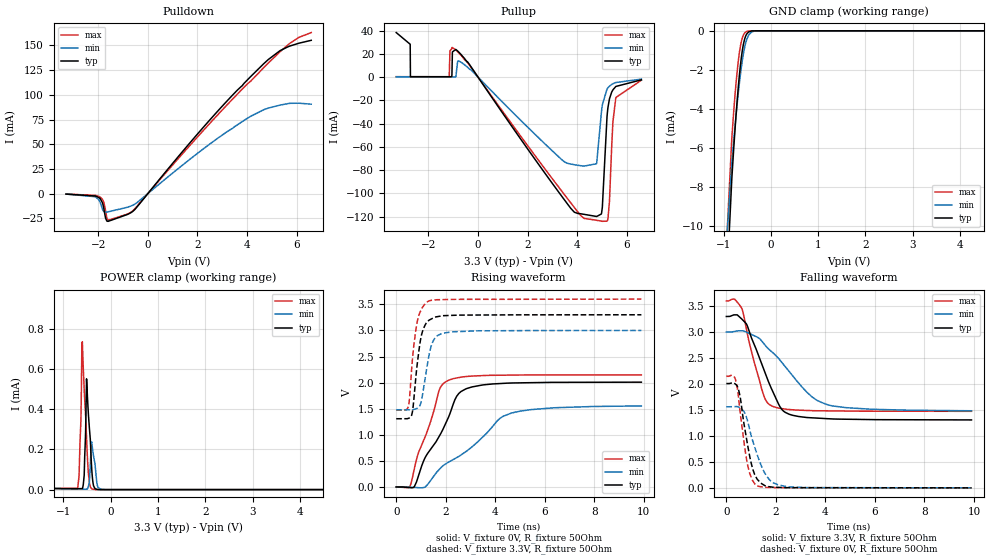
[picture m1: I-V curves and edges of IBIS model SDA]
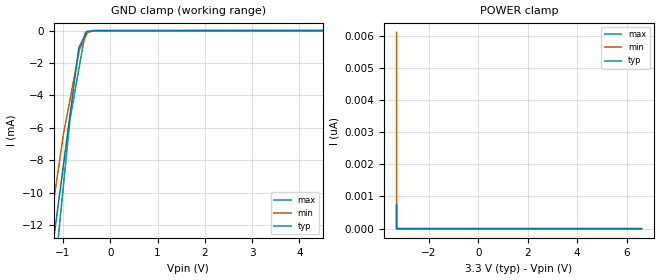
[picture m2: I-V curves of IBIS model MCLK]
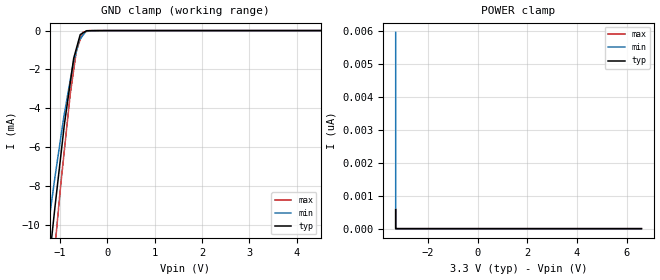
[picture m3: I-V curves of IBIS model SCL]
| Texas Instruments Incorporated
| 25-W STEREO AMPLIFIER WITH EQ, DRC, AND DIRECT-PATH HEADPHONE AMPLIFIER
| Marketing part#   Voltage Range   Package-type   #pins/pkg drawing
| TAS5729MD   3.0V - 3.6V   TQFP   48-pin TQFP
[IBIS Ver]   4.0
[File name]   tas5729md.ibs
[File Rev]   1.0
[Date]   06/06/2012
[Source]   Model built from TISPICED simulations at:
   Texas Instruments Incorporated.
   Analog-eLab, HPA
   12500 TI Blvd
   Dallas, TX -75243
   For Support e-mail: elab_ibis@list.ti.com
[Notes]   Revision History
   Rev 1.0: 06/06/2012
   - ccomp values are based on PVT settings:
   WEAK: Low Voltage, High Temperature, Weak Process
   NOM: Nominal Voltage, Nominal Temperature, Nominal Process
   STRONG: High Voltage, Low Temperature, Fast Process
   - User may change ccomp in the order of number values as
   per end simulator used
   - C_comp although listed in numberical order of value are obtained from varying PVT conditions.
   For PVT conditions for each specific value, refer to the buffer description under repective [Model].
   IBIS model user is responsible for using appropriate C_comp to simulate for Signal Integrity.
   - Non-monotonic behavior in SDA model is a result of simulation.
[Disclaimer] This model is designed as an aid for customers of Texas Instruments.
 TI and its licensors and suppliers make no warranties, either expressed
 or implied, with respect to this  model, including the warranties of
 merchantability or fitness for a particular purpose.
 The model is provided solely on an "as is" basis. The entire risk as to
 its quality and performance is with the customer.
[Copyright] (C)Copyright 2012 Texas Instruments Incorporated.
   All rights reserved.
|   Component TAS5729MD
[Component]   TAS5729MD
[Manufacturer]  Texas Instruments Incorporated
[Package]   |48-pin TQFP PHP package
|   typ   min   max
R_pkg   0.111   0.052   0.195
L_pkg   2.811nH   1.641nH   4.365nH
C_pkg   0.561pF   0.383pF   0.971pF
[Pin] signal_name   model_name   R_pin   L_pin   C_pin
1   GND   GND   0.06305   3.25293nH   0.9711pF
2   OUTA   NC   0.08589   3.49122nH   0.77876pF
3   BSTA   NC   0.16148   3.75361nH   0.72245pF
4   PVDD   POWER   0.06585   2.58699nH   0.74279pF
5   PWM1   NC   0.07479   2.04281nH   0.58008pF
6   PWM2   NC   0.06489   1.79675nH   0.55462pF
7   HPIL   NC   0.06029   1.67272nH   0.54983pF
8   HPOL   NC   0.06108   1.65283nH   0.5297pF
9   HPOR   NC   0.06399   1.64098nH   0.52278pF
10   HPIR   NC   0.06787   1.70652nH   0.54865pF
11   HPVSS   NC   0.07197   1.75312nH   0.54261pF
12   CN   NC   0.14722   2.80415nH   0.40929pF
13   CP   NC   0.16145   3.02753nH   0.43109pF
14   HPVDD   NC   0.17406   3.23001nH   0.45908pF
15   GND   GND   0.06558   2.05127nH   0.44725pF
16   FLTM   NC   0.1246   2.46433nH   0.42269pF
17   FTLP   NC   0.13785   2.72862nH   0.45429pF
18   AVDD_REG1   NC   0.15617   3.04909nH   0.4946pF
19   AVDD   POWER   0.09525   3.06484nH   0.55645pF
20   ADR   SDIN   0.19547   3.8041nH   0.50443pF
21   MCLK   MCLK   0.14557   3.25076nH   0.56537pF
22   ROSC   NC   0.14501   3.50685nH   0.71349pF
23   GND   GND   0.09037   3.53737nH   0.80119pF
24   DVDD_REG   NC   0.10021   4.1032nH   0.7864pF
25   PDN   SDIN   0.15766   4.36474nH   0.75795pF
26   LRCLK   MCLK   0.15465   3.95793nH   0.77612pF
27   SCLK   MCLK   0.1548   3.65915nH   0.72538pF
28   SDIN1   SDIN   0.15922   3.46366nH   0.58952pF
29   SDA   SDA   0.15909   3.2297nH   0.47015pF
30   SCLK   SCL   0.13875   2.82626nH   0.47213pF
31   NC   NC   0.01329   1.07519nH   0.34093pF
32   RESET   NC   0.10958   2.28802nH   0.41439pF
33   TEST   SDIN   0.1143   2.30153nH   0.40259pF
34   DVDD_REG   NC   0.06503   2.0377nH   0.45379pF
35   GND   GND   0.06927   2.14655nH   0.4476pF
36   GND   GND   0.0667   2.76518nH   0.50798pF
37   AVDD_REG2   NC   0.13522   2.61575nH   0.39962pF
38   SSTIMER   NC   0.11443   2.29623nH   0.40178pF
39   HP_SD   SDIN   0.09788   2.05796nH   0.39429pF
40   GVDD_REG   NC   0.09356   1.98511nH   0.38289pF
41   PVDD   POWER   0.05208   1.71793nH   0.43123pF
42   BSTD   NC   0.12894   2.61575nH   0.44892pF
43   OUTD   NC   0.06255   2.07268nH   0.45804pF
44   GND   GND   0.07388   2.51643nH   0.47374pF
45   OUTC   NC   0.08514   3.06822nH   0.60309pF
46   BSTC   NC   0.17429   3.95481nH   0.73604pF
47   BSTB   NC   0.17257   4.22889nH   0.78027pF
48   OUTB   NC   0.0948   3.99nH   0.77185pF
| Models and submodels in the file (4): SDA (I/O), MCLK (Input), SCL (Input), SDIN (Input)
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[Model]   SDA
Model_type   I/O
Polarity   Non-Inverting
Vinl = 0.8
Vinh = 2.0
Vmeas = 1.65
Vref = 1.65
Cref = 15pF
Rref = 50
|   typ   min   max
C_comp   0.7443p   0.7440p   0.7473p
[Voltage Range]   3.3   3   3.6
[Temperature Range]   27   125   0
[Pullup Reference]   3.3   3   3.6
[Pulldown Reference]   -0   -0   -0
[Power Clamp Reference]   3.3   3   3.6
[GND Clamp Reference]   -0   -0   -0
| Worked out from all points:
|   slope of the pulldown table from 0 to 0.495 V, typ, clamps not added: 32.5 ohm
|   slope of the pullup table from 0 to 0.495 V, typ, clamps not added: 31.9 ohm
|   GND clamp passes 1 mA (typ) near -0.60 V on its own axis
|   POWER clamp passes 1 mA (typ) near -3.29 V on its own axis
|   falling waveform, V_fixture 3.3V, R_fixture 50Ohm: 20-80 % time 1.01ns typ, 1.72ns min, 668ps max; typ from 3.3 V to 1.31 V
|   rising waveform, V_fixture 0V, R_fixture 50Ohm: 20-80 % time 1.29ns typ, 2.35ns min, 888ps max; typ from 0 V to 2.01 V
|   rising waveform, V_fixture 3.3V, R_fixture 50Ohm: 20-80 % time 299ps typ, 342ps min, 283ps max; typ from 1.31 V to 3.3 V
|   falling waveform, V_fixture 0V, R_fixture 50Ohm: 20-80 % time 440ps typ, 642ps min, 368ps max; typ from 2.01 V to 0 V
[Pulldown]
|   Voltage   I(typ)   I(min)   I(max)
-3.3V     -559.9uA   -542.7uA   -469.7uA
-2.122V   -2.468mA   -3.204mA   -1.888mA
-1.983V   -3.945mA   -6.17mA    -2.853mA
-1.785V   -14.05mA   -17.97mA   -8.449mA
-1.706V   -24.93mA   -18.84mA   -17.74mA
-1.637V   -28.06mA   -18.67mA   -26.01mA
-686.4mV  -19.39mA   -12.65mA   -19.01mA
2.363V    70.7mA     47.61mA    67.34mA
4.155V    118.7mA    78.38mA    114mA
5.333V    144.8mA    89.61mA    143.7mA
6.095V    152.3mA    91.5mA     158.2mA
6.59V     155.2mA    90.54mA    163.1mA
[GND Clamp]
|   Voltage   I(typ)   I(min)   I(max)
-3.3V     -1.514A    -1.357A    -1.56A
-1.607V   -47.21mA   -35.03mA   -43.52mA
-825mV    -7.581mA   -6.783mA   -5.501mA
-745.8mV  -4.664mA   -4.596mA   -2.961mA
-706.2mV  -3.403mA   -3.61mA    -1.948mA
-666.6mV  -2.316mA   -2.718mA   -1.15mA
-627mV    -1.437mA   -1.937mA   -591.7uA
-587.4mV  -790.1uA   -1.288mA   -259.8uA
-508.2mV  -156.3uA   -434.6uA   -32.58uA
-409.2mV  -10.58uA   -65.64uA   -1.24uA
-270.6mV  -46.46nA   -2.385uA   0A
6.59V     0A         0A         0A
[Pullup]
|   Voltage   I(typ)   I(min)   I(max)
-3.3V     38.34mA    165.8uA    389.7uA
-2.736V   28.28mA    154uA      344uA
-2.726V   348.7uA    153.8uA    343.5uA
-1.162V   326.1uA    144.3uA    317.2uA
-1.063V   357.5uA    144.2uA    24.35mA
-894.3mV  23.79mA    154.1uA    23.32mA
4.026V    -117.4mA   -75.91mA   -116mA
4.778V    -119.9mA   -74.6mA    -123.2mA
4.976V    -117.8mA   -30.66mA   -124mA
5.224V    -29.62mA   -9.709mA   -123.2mA
5.561V    -8.046mA   -4.65mA    -17.58mA
6.59V     -2.35mA    -1.735mA   -2.682mA
[POWER Clamp]
|   Voltage   I(typ)   I(min)   I(max)
-3.3V     1.038mA    9.254mA    692.2uA
-2.874V   479.6uA    1.182mA    323.7uA
-2.627V   255.8uA    434.3uA    140.4uA
-2.023V   7.025uA    93.11uA    6.497uA
-696.3mV  4.878uA    2.32uA     6.22uA
-627mV    4.868uA    2.316uA    346.2uA
-597.3mV  4.824uA    2.315uA    736.5uA
-557.7mV  72.19uA    2.312uA    496.7uA
-508.2mV  551.7uA    2.308uA    257.9uA
-389.4mV  71.88uA    217.3uA    3.215uA
-211.2mV  69.71nA    2.032uA    0A
6.59V     0A         0A         0A
[Ramp]
R_load = 50
|   typ   min   max
dV/dt_r   1.20505/1.28979e-09   0.932073/2.35176e-09   1.28889/8.87513e-10
dV/dt_f   1.1951/1.01652e-09   0.909529/1.72053e-09   1.27543/6.67234e-10
[Falling Waveform]
V_fixture = 3.3V
V_fixture_min = 3V
V_fixture_max = 3.6V
R_fixture = 50Ohm
C_fixture = 0F
|   Time   V(typ)   V(min)   V(max)
0s        3.3V       3V         3.6V
332.3ps   3.331V     3.012V     3.634V
631.3ps   3.247V     3.024V     3.448V
830.9ps   3.138V     2.994V     3.012V
1.472ns   2.334V     2.803V     1.834V
1.851ns   1.881V     2.614V     1.574V
2.371ns   1.456V     2.339V     1.517V
3.451ns   1.349V     1.755V     1.487V
4.086ns   1.332V     1.601V     1.483V
9.9ns     1.308V     1.484V     1.474V
[Rising Waveform]
V_fixture = 0V
V_fixture_min = 0V
V_fixture_max = 0V
R_fixture = 50Ohm
C_fixture = 0F
|   Time   V(typ)   V(min)   V(max)
0s        951pV      57.66nV    -337.4nV
565.5ps   -13.03mV   -3.808mV   23.65mV
730.3ps   4.516mV    -8.506mV   343.5mV
1.146ns   541.2mV    -6.853mV   936.5mV
1.742ns   976.2mV    337.4mV    1.863V
2.078ns   1.301V     466.5mV    2.037V
2.371ns   1.673V     543.9mV    2.083V
2.615ns   1.828V     613.4mV    2.105V
4.634ns   1.992V     1.413V     2.144V
9.9ns     2.008V     1.553V     2.148V
[Rising Waveform]
V_fixture = 3.3V
V_fixture_min = 3V
V_fixture_max = 3.6V
R_fixture = 50Ohm
C_fixture = 0F
|   Time   V(typ)   V(min)   V(max)
0s        1.308V     1.479V     1.474V
467.9ps   1.312V     1.478V     1.512V
541.1ps   1.326V     1.477V     1.722V
622.6ps   1.374V     1.48V      2.249V
816.5ps   2.216V     1.502V     3.08V
984.4ps   2.827V     1.593V     3.372V
1.318ns   3.193V     2.506V     3.564V
1.541ns   3.25V      2.838V     3.583V
2.058ns   3.286V     2.96V      3.593V
9.9ns     3.3V       3V         3.6V
[Falling Waveform]
|Gnd
V_fixture = 0V
V_fixture_min = 0V
V_fixture_max = 0V
R_fixture = 50Ohm
C_fixture = 0F
|   Time   V(typ)   V(min)   V(max)
0s        2.009V     1.56V      2.148V
325.6ps   2.014V     1.564V     2.132V
475.2ps   1.918V     1.56V      1.812V
715ps     1.228V     1.467V     874.5mV
849.4ps   850.4mV    1.304V     465.1mV
1.047ns   395.2mV    934.3mV    155.2mV
1.256ns   160.8mV    625.9mV    37.79mV
1.755ns   20.76mV    150.1mV    8.108mV
2.528ns   3.802mV    17.6mV     2.766mV
9.9ns     21.89uV    142.1uV    -337.4nV
[Model]   MCLK
Model_type   Input
Vinl = .8
Vinh = 2
|   typ   min   max
C_comp   0.7443p   0.7440p   0.7473p
[Voltage Range]   3.3   3   3.6
[Temperature Range]   27   125   0
[Power Clamp Reference]   3.3   3   3.6
[GND Clamp Reference]   -0   -0   -0
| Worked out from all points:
|   GND clamp passes 1 mA (typ) near -0.65 V on its own axis
[GND Clamp]
|   Voltage   I(typ)   I(min)   I(max)
-3.3V     -1.514A    -1.357A    -1.56A
-1.441V   -19.09mA   -15.41mA   -22.82mA
-1.238V   -13.78mA   -11.35mA   -16.83mA
-988.3mV  -8.243mA   -6.357mA   -9.481mA
-852.9mV  -5.236mA   -4.277mA   -5.487mA
-665.8mV  -1.08mA    -1.402mA   -2.396mA
-649.3mV  -979.8uA   -1.149mA   -2.125mA
-529.9mV  -249.7uA   -419.5uA   -152.6uA
-497.8mV  -53.24uA   -223uA     -123.4uA
-358.6mV  -12.14uA   -10.45uA   -5.776uA
-237.4mV  -3.461uA   -2.36uA    -4.816uA
6.6V      0A         0A         0A
[POWER Clamp]
|   Voltage   I(typ)   I(min)   I(max)
-3.3V     728.6pA    6.099nA    754.7pA
-3.3V     0A         0A         0A
-3.3V     0A         0A         0A
6.6V      0A         0A         0A
[Model]   SCL
Model_type   Input
Vinl = .8
Vinh = 2
|   typ   min   max
C_comp   0.7443p   0.7440p   0.7473p
[Voltage Range]   3.3   3   3.6
[Temperature Range]   27   125   0
[Power Clamp Reference]   3.3   3   3.6
[GND Clamp Reference]   -0   -0   -0
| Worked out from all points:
|   GND clamp passes 1 mA (typ) near -0.66 V on its own axis
[GND Clamp]
|   Voltage   I(typ)   I(min)   I(max)
-3.3V     -1.514A    -1.356A    -1.56A
-1.372V   -15.31mA   -12.42mA   -18.38mA
-1.237V   -12.18mA   -9.983mA   -14.75mA
-1.157V   -10.35mA   -8.537mA   -12.59mA
-1.102V   -9.096mA   -7.552mA   -11.15mA
-904.1mV  -4.85mA    -4.296mA   -6.176mA
-780.4mV  -2.711mA   -2.57mA    -3.29mA
-706.1mV  -1.425mA   -1.591mA   -2.019mA
-648.3mV  -913.9uA   -1.062mA   -1.032mA
-516.3mV  -130.2uA   -261uA     -91.17uA
-320.4mV  -5.141uA   -2.758uA   -960.6nA
6.6V      0A         0A         0A
[POWER Clamp]
|   Voltage   I(typ)   I(min)   I(max)
-3.3V     572.5pA    5.955nA    588.9pA
-3.3V     0A         0A         0A
-3.3V     0A         0A         0A
6.6V      0A         0A         0A
